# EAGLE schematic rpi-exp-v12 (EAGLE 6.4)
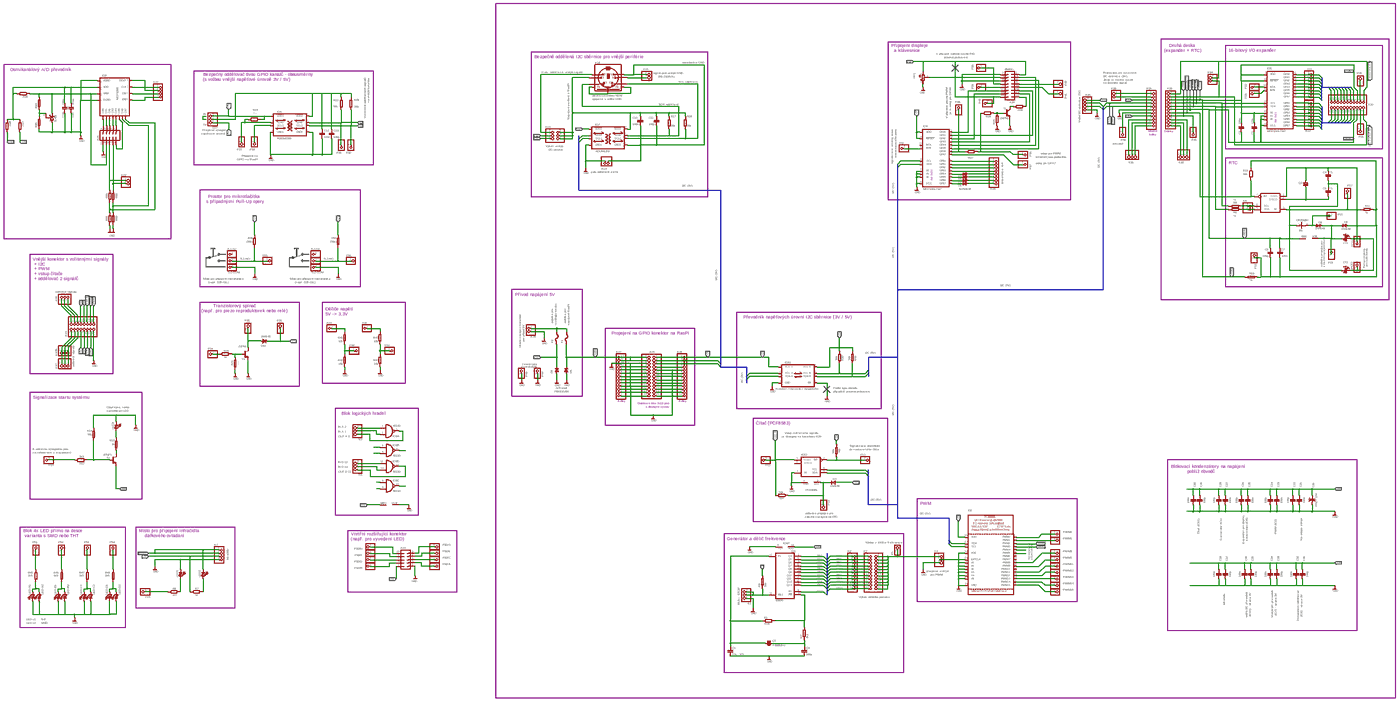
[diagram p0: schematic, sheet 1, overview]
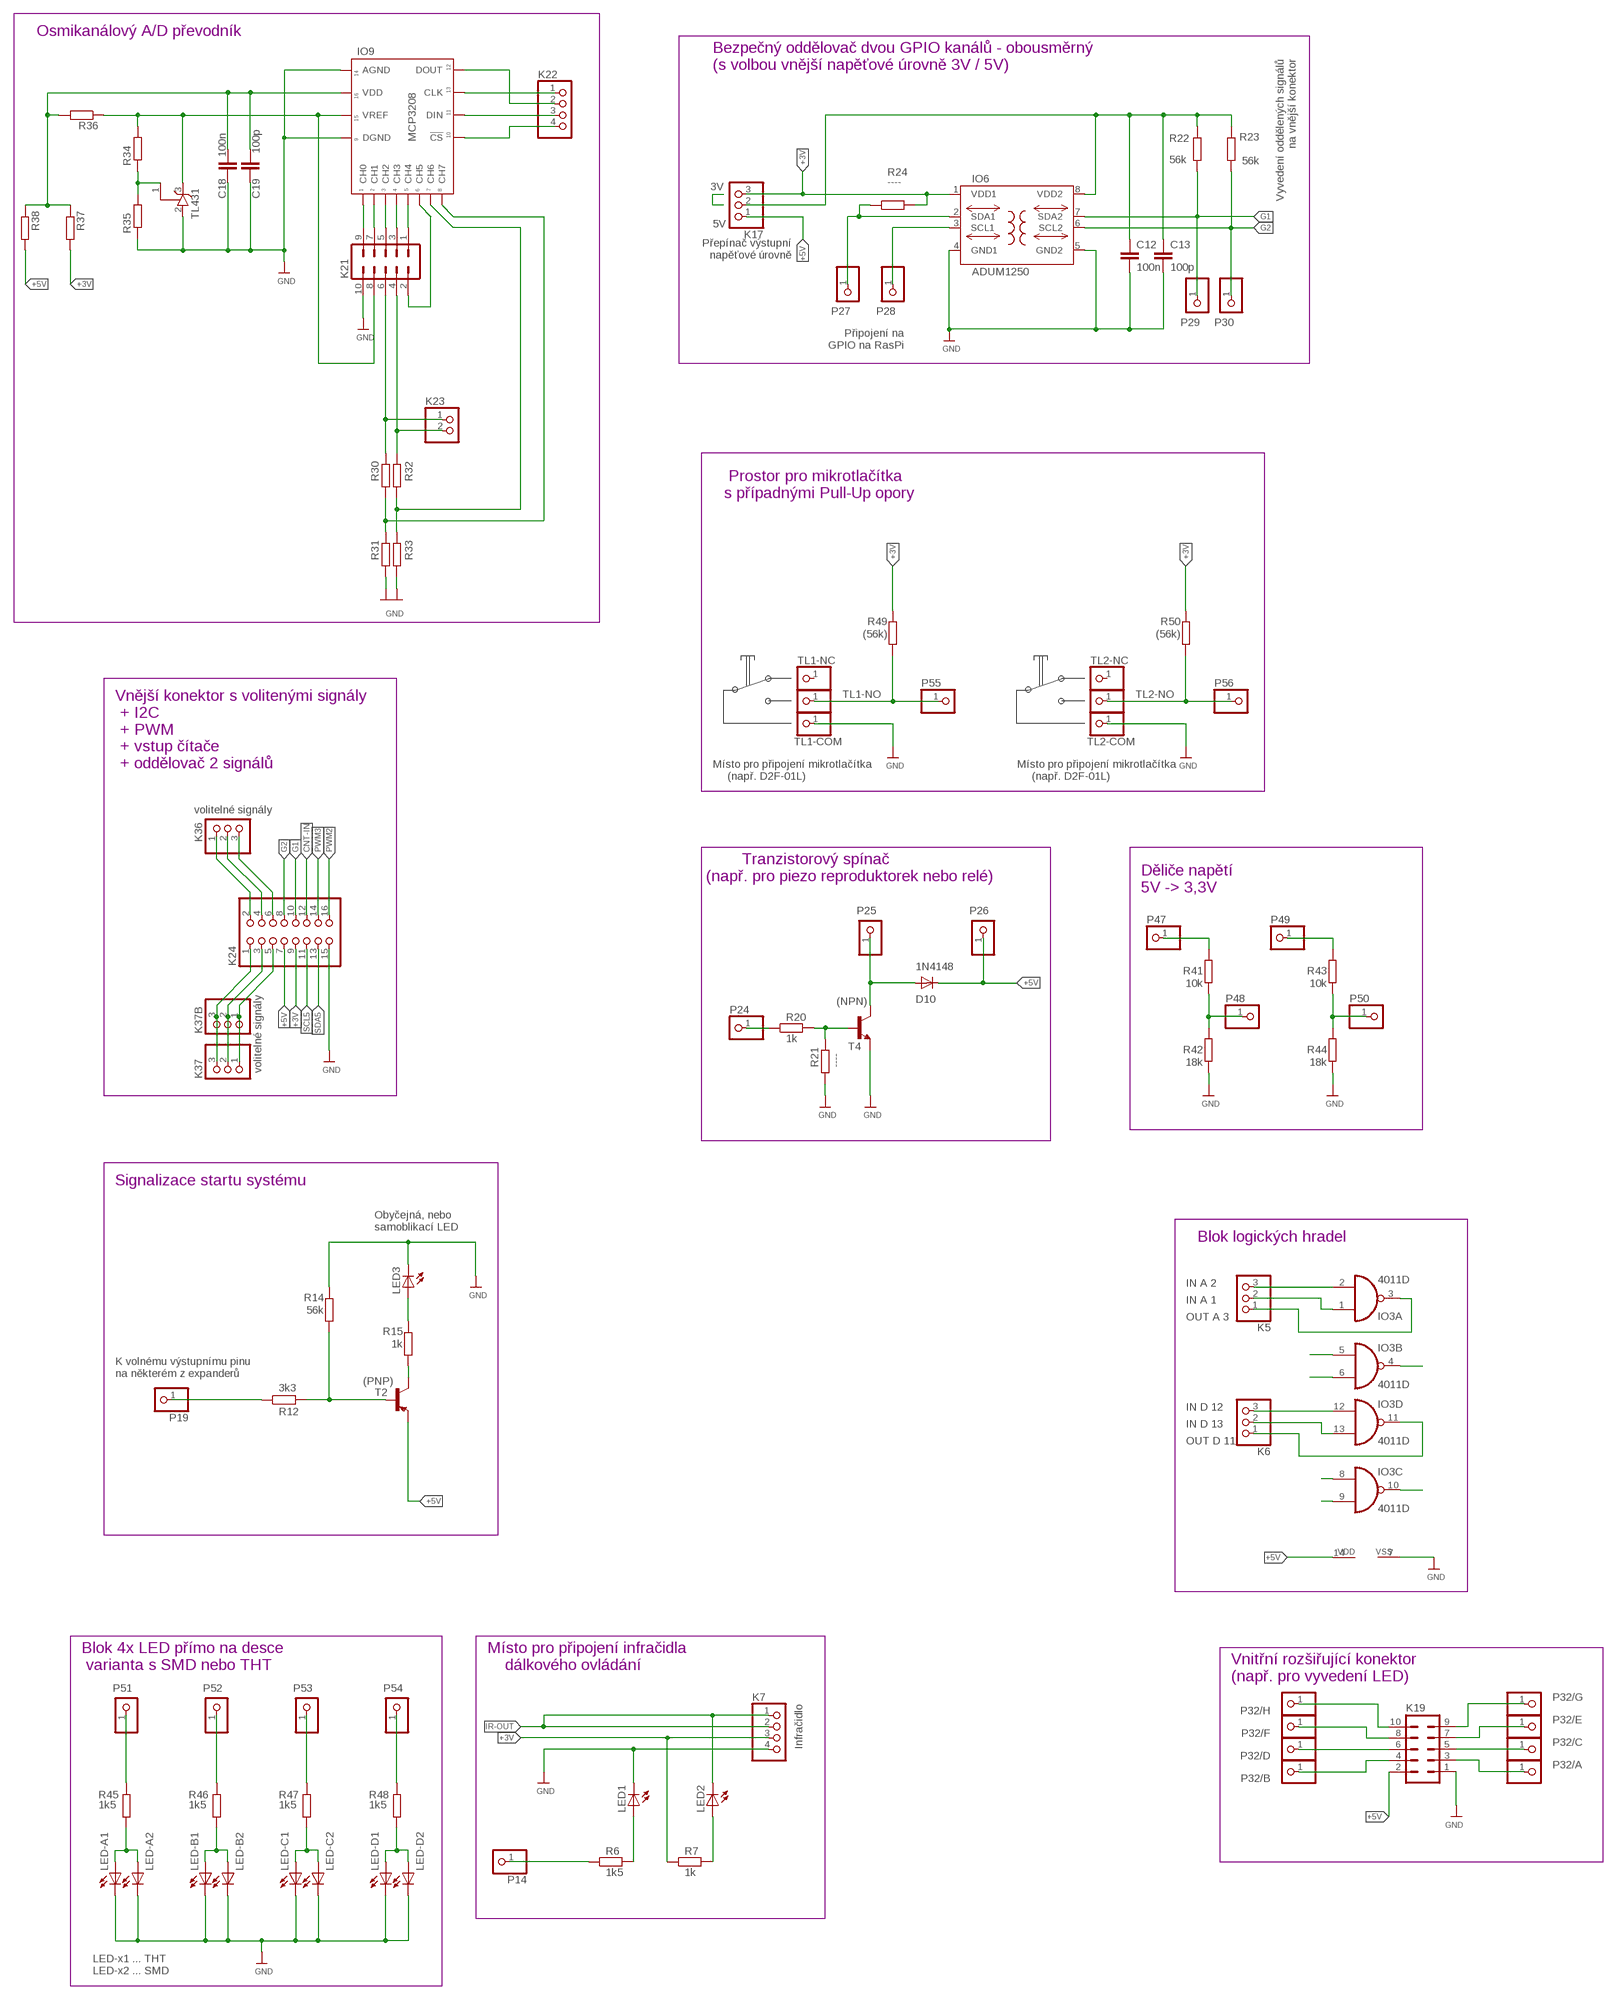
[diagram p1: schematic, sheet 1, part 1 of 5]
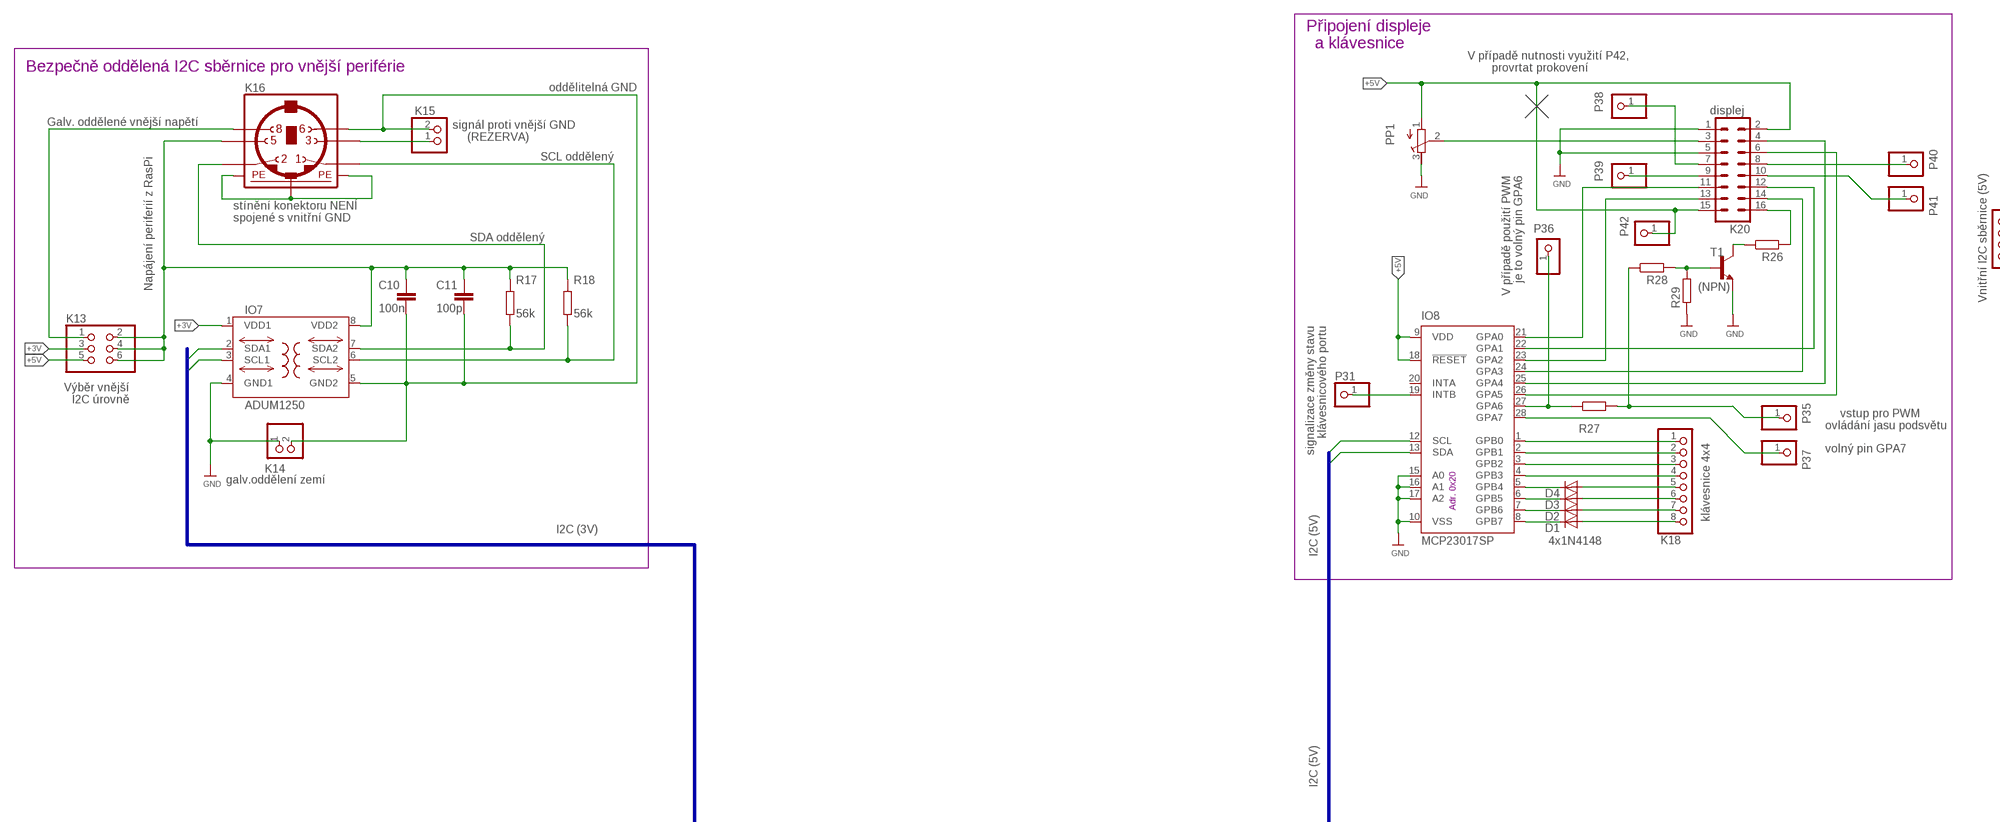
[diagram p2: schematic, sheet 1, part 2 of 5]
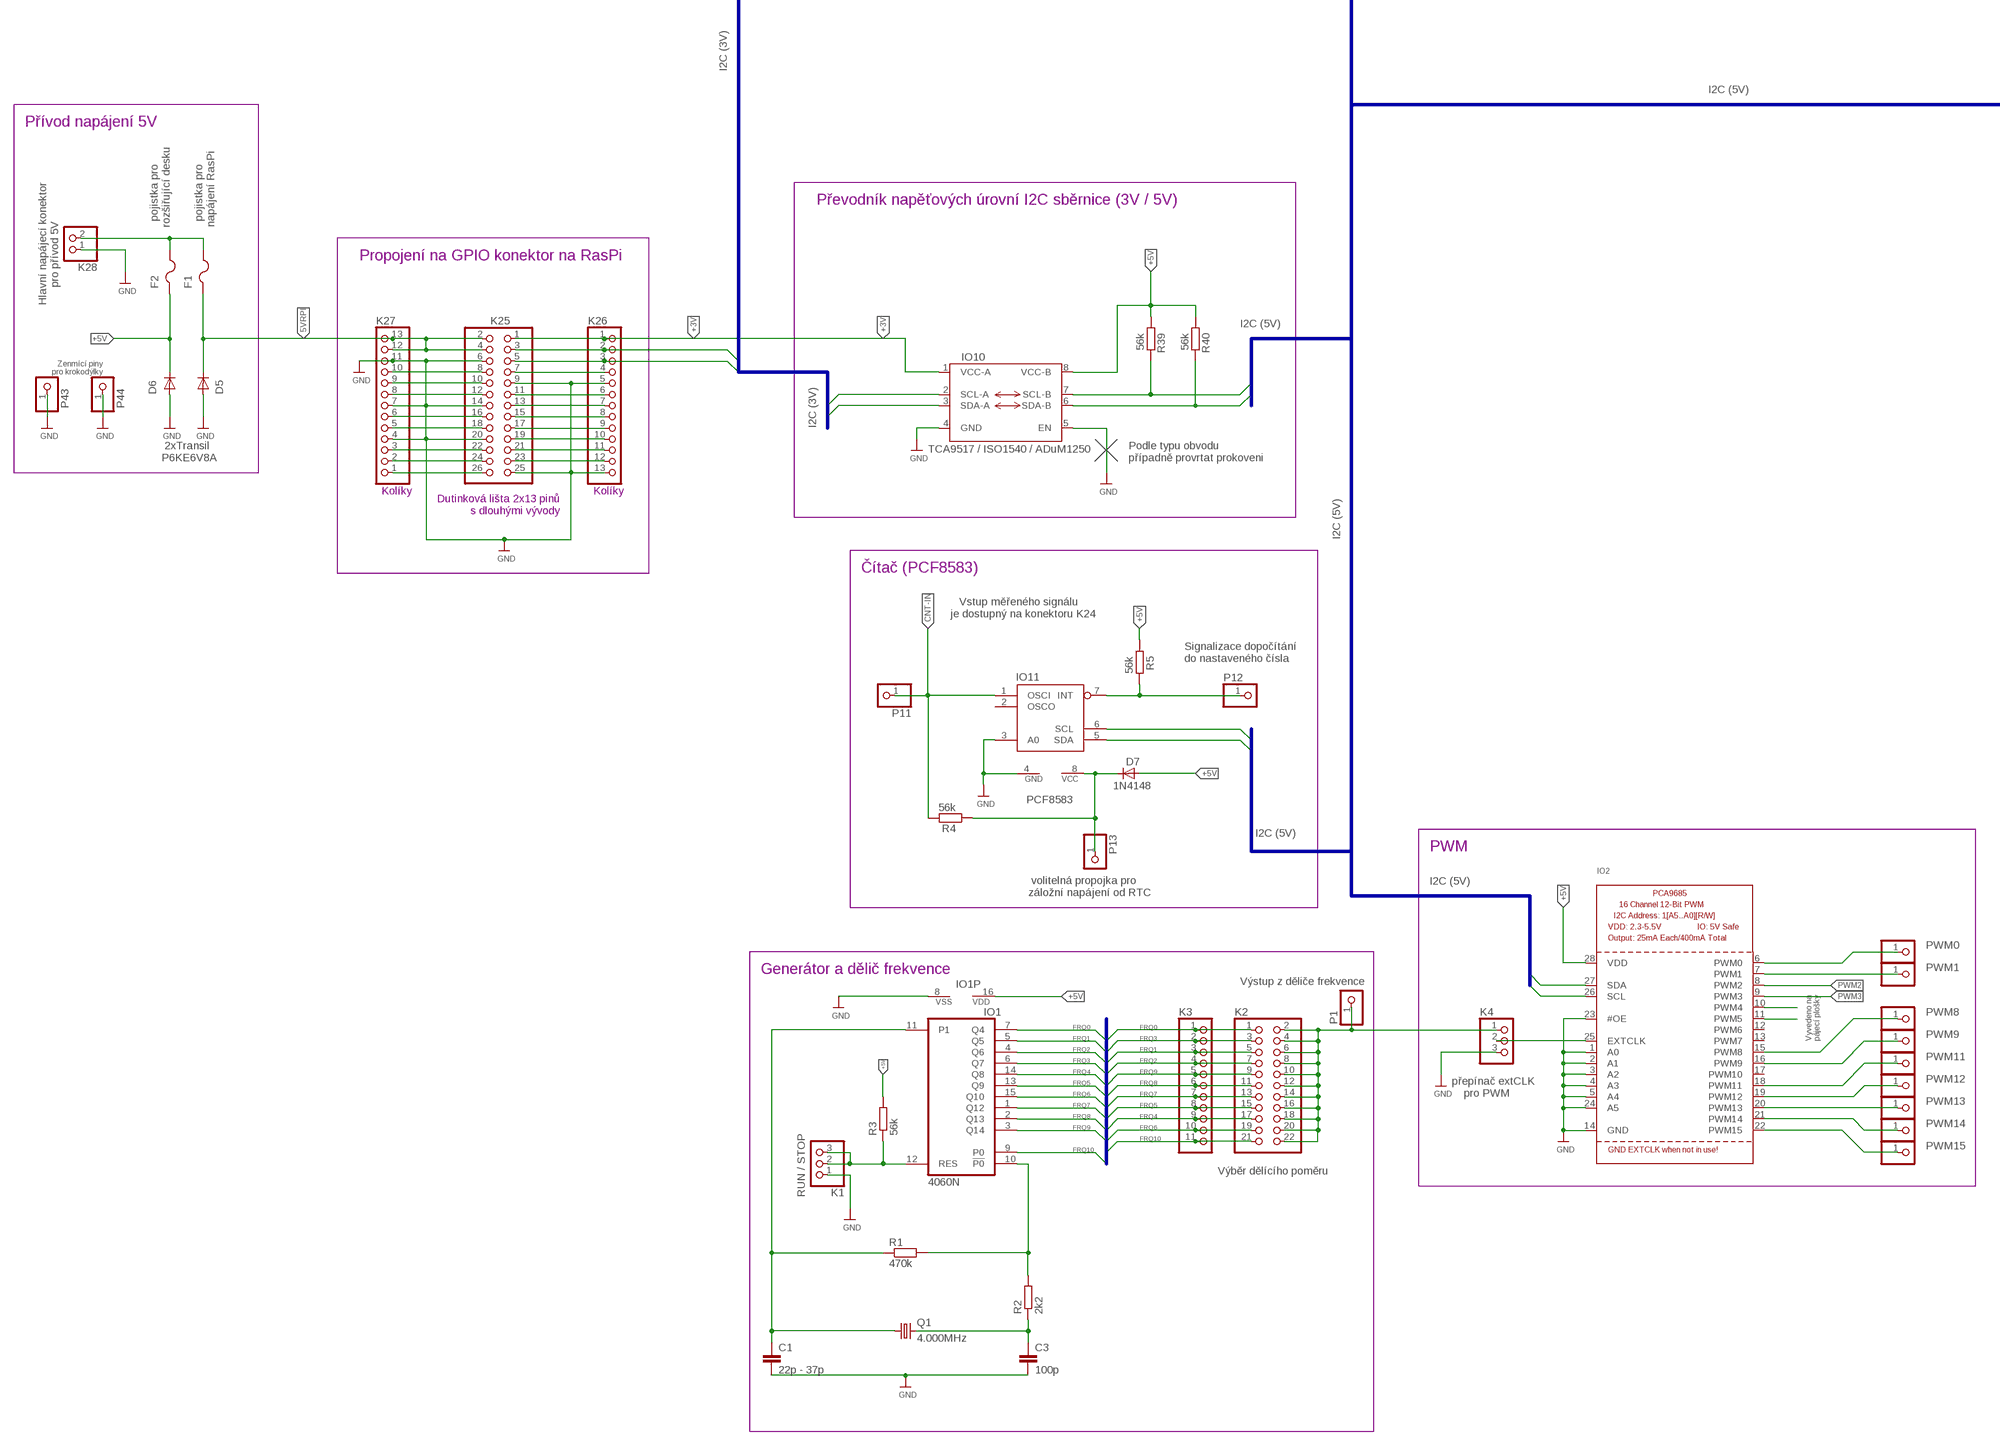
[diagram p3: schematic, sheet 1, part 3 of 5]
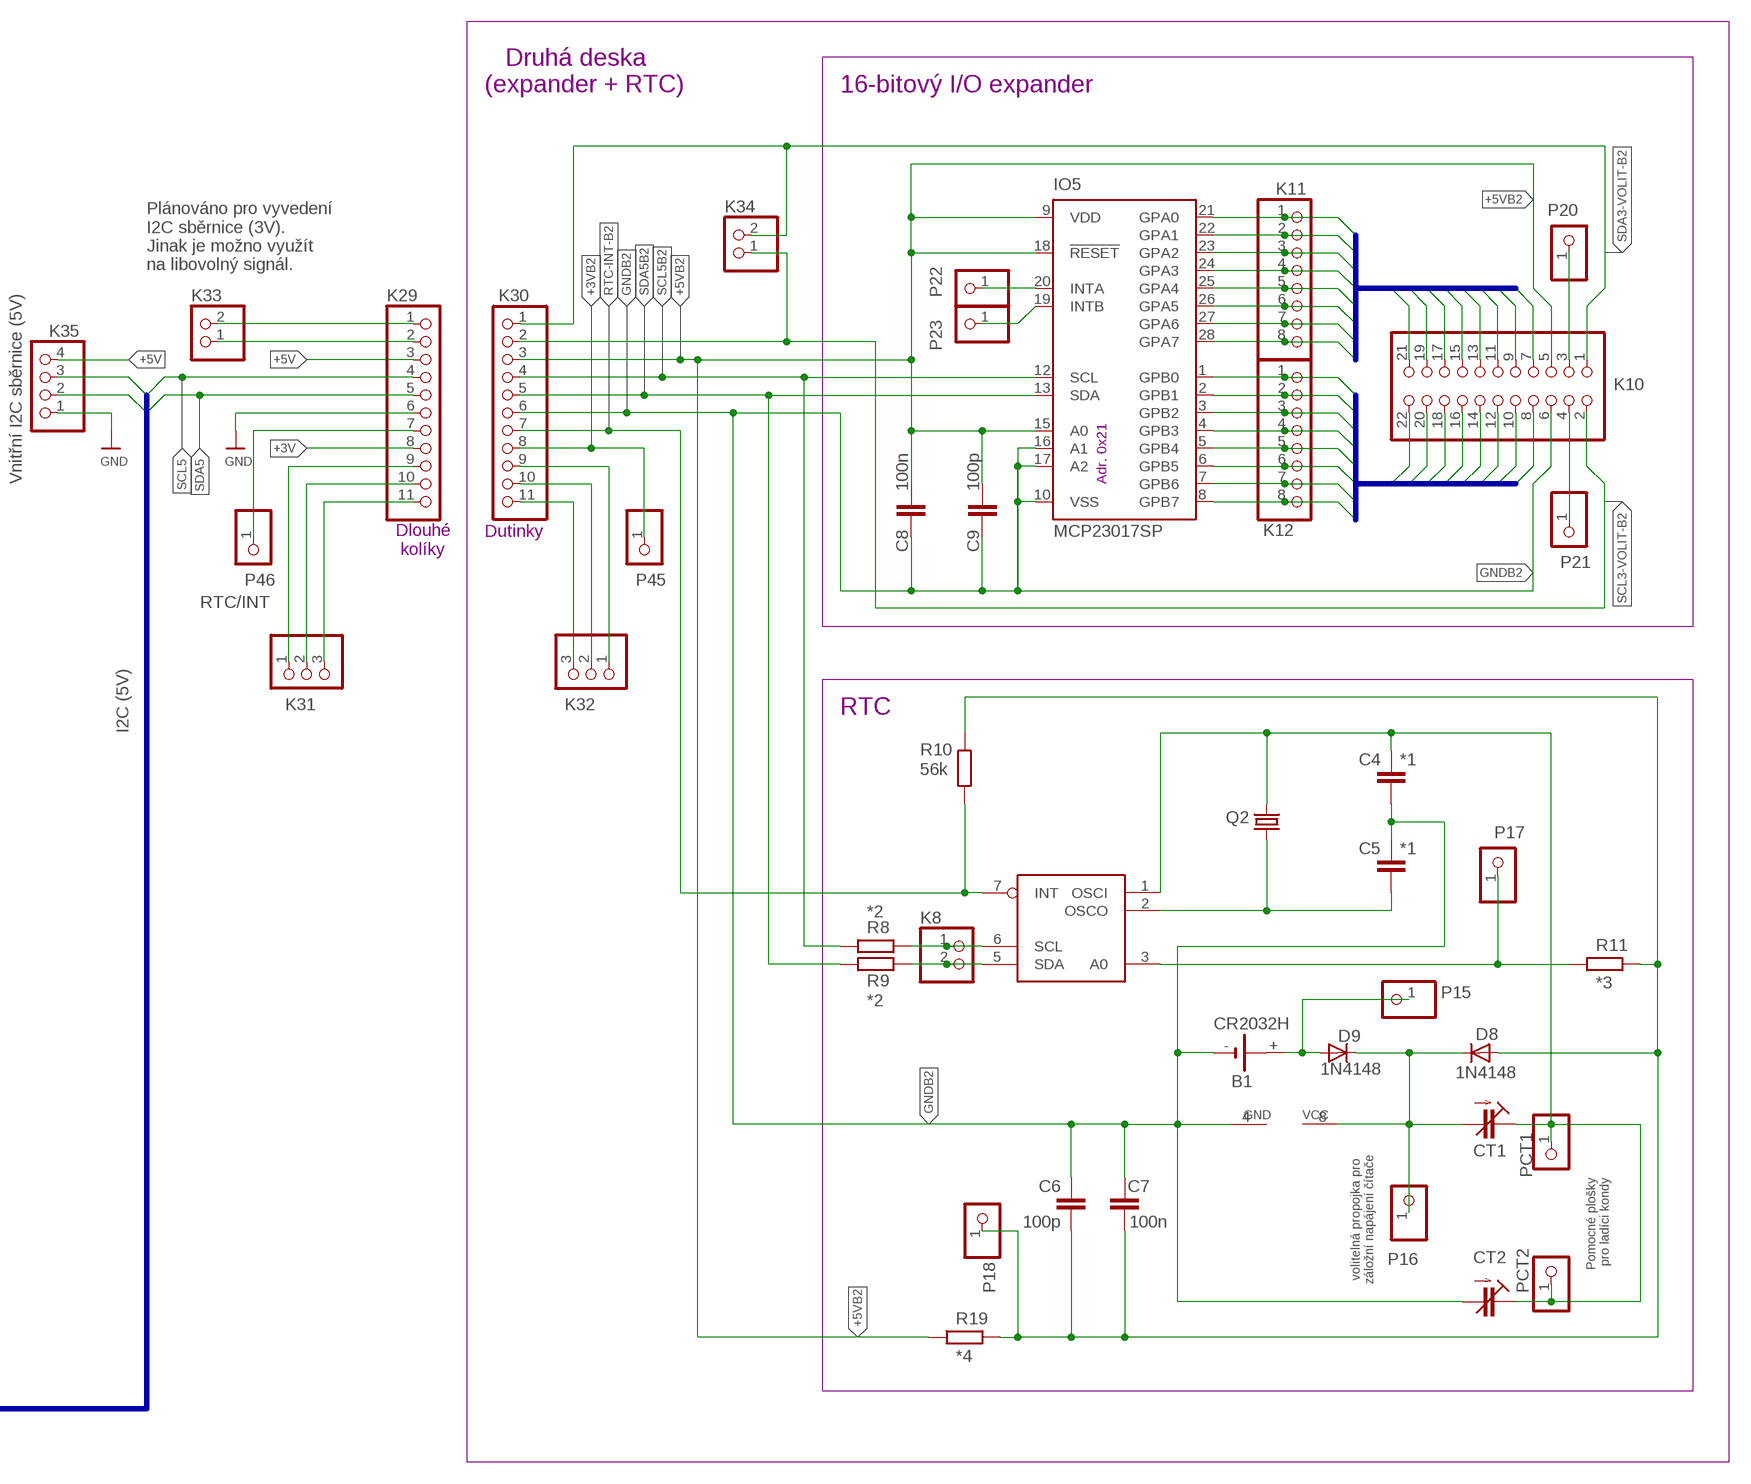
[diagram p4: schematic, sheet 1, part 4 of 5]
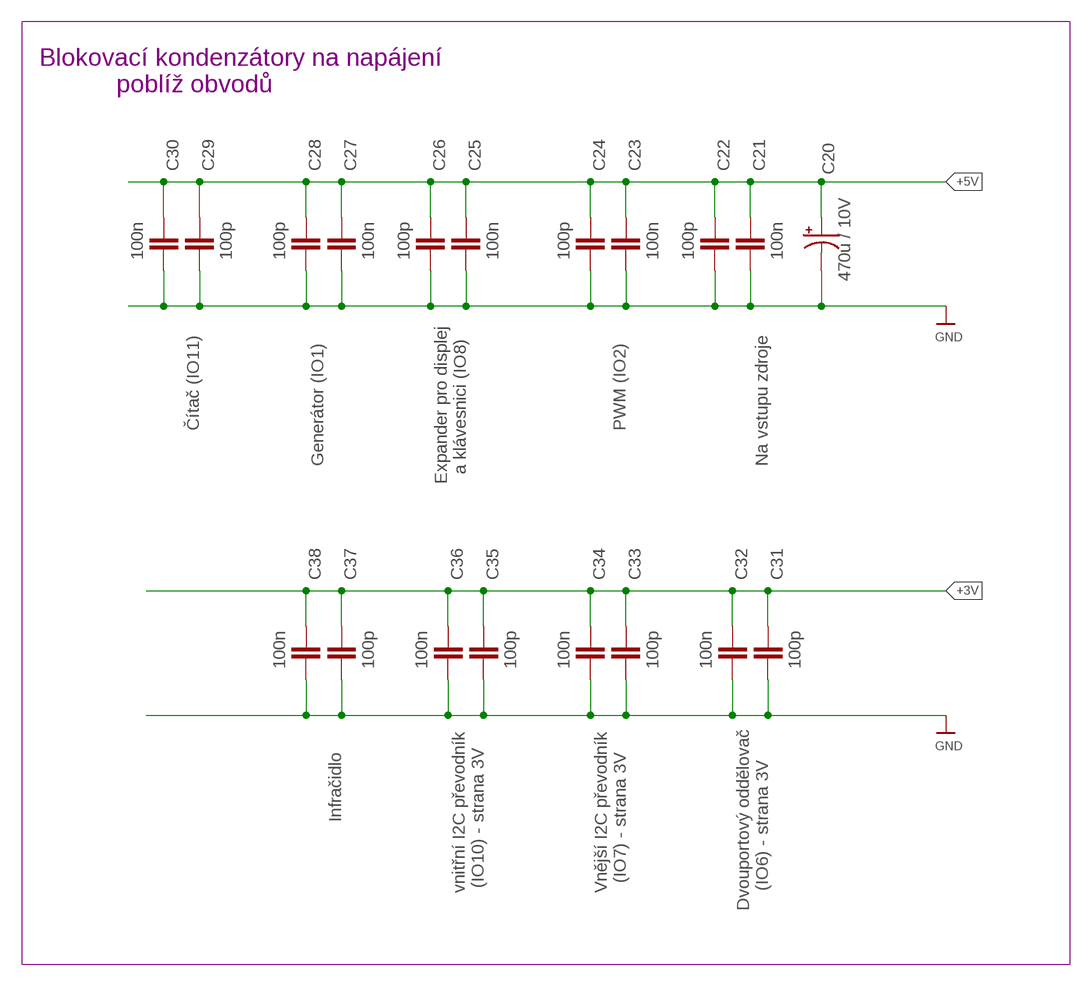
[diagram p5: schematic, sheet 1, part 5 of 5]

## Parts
B1  CR2032H  [CR2032H]
C1  22p - 37p  C-SMD0805  [0805]
C3  100p  C-SMD0805  [0805]
C4  *1  C-SMD0805  [0805]
C5  *1  C-SMD0805  [0805]
C6  100p  C-SMD0805  [0805]
C7  100n  C-SMD0805  [0805]
C8  100n  C-SMD0805  [0805]
C9  100p  C-SMD0805  [0805]
C10  100n  C-SMD0805  [0805]
C11  100p  C-SMD0805  [0805]
C12  100n  C-SMD0805  [0805]
C13  100p  C-SMD0805  [0805]
C18  100n  C-SMD0805  [0805]
C19  100p  C-SMD0805  [0805]
C20  470u / 10V  CPOL-USE5-8.5  [E5-8,5]
C21  100n  C-SMD0805  [0805]
C22  100p  C-SMD0805  [0805]
C23  100n  C-SMD0805  [0805]
C24  100p  C-SMD0805  [0805]
C25  100n  C-SMD0805  [0805]
C26  100p  C-SMD0805  [0805]
C27  100n  C-SMD0805  [0805]
C28  100p  C-SMD0805  [0805]
C29  100p  C-SMD0805  [0805]
C30  100n  C-SMD0805  [0805]
C31  100p  C-SMD0805  [0805]
C32  100n  C-SMD0805  [0805]
C33  100p  C-SMD0805  [0805]
C34  100n  C-SMD0805  [0805]
C35  100p  C-SMD0805  [0805]
C36  100n  C-SMD0805  [0805]
C37  100p  C-SMD0805  [0805]
C38  100n  C-SMD0805  [0805]
CT1  C-TRIMM3040.427  [CTRIM3040.427]
CT2  C-TRIMM3040.427  [CTRIM3040.427]
D1  1N4148  DIODE-SOD106A-R  [SOD106A-R]
D2  1N4148  DIODE-SOD106A-R  [SOD106A-R]
D3  1N4148  DIODE-SOD106A-R  [SOD106A-R]
D4  1N4148  DIODE-SOD106A-R  [SOD106A-R]
D5  P6KE6V8A  1N4004  [DO41-10]
D6  P6KE6V8A  1N4004  [DO41-10]
D7  1N4148  D-SOD-80  [SOD80]
D8  1N4148  D-SOD-80  [SOD80]
D9  1N4148  D-SOD-80  [SOD80]
D10  1N4148  DIODE-SOD106A-R  [SOD106A-R]
F1  PTCFUSE-1812  [1812]
F2  PTCFUSE-1812  [1812]
I04  PCF8583P  [DIL08]
IO1  4060N  [DIL16]
IO2  PCA9685  [TSSOP28]
IO3  4011D  [SO14]
IO5  MCP23017SP  [DIL28-3]
IO6  ADUM1250  [SO8-COOL]
IO7  ADUM1250  [SO8-COOL]
IO8  MCP23017SP  [DIL28-3]
IO9  MCP3208  21298EDIP  [DIP16]
IO10  TCA9517 / ISO1540 / ADuM1250  TCA9517  [SO8-COOL]
IO11  PCF8583P  [DIL08]
K1  PINHD-1X3  [1X03]
K2  PINHD-2X11  [2X11]
K3  PINHD-1X11  [1X11]
K4  PINHD-1X3  [1X03]
K5  PINHD-1X3  [1X03]
K6  PINHD-1X3  [1X03]
K7  PINHD-1X4  [1X04]
K8  PINHD-1X2  [1X02]
K10  PINHD-2X11/90  [2X11/90]
K11  PINHD-1X8  [1X08]
K12  PINHD-1X8  [1X08]
K13  PINHD-2X3  [2X03]
K14  PINHD-1X2  [1X02]
K15  PINHD-1X2  [1X02]
K16  MINI_DIN_6  [M_DIN6]
K17  PINHD-1X3  [1X03]
K18  PINHD-1X8  [1X08]
K19  ML10  [ML10]
K20  ML16  [ML16]
K21  ML10L  [ML10L]
K22  PINHD-1X4  [1X04]
K23  PINHD-1X2  [1X02]
K24  PINHD-2X8/90  [2X08/90]
K25  PINHD-2X13  [2X13]
K26  PINHD-1X13  [1X13]
K27  PINHD-1X13  [1X13]
K28  PINHD-1X2  [1X02]
K29  PINHD-1X11  [1X11]
K30  PINHD-1X11  [1X11]
K31  PINHD-1X3  [1X03]
K32  PINHD-1X3  [1X03]
K33  PINHD-1X2  [1X02]
K34  PINHD-1X2  [1X02]
K35  PINHD-1X4  [1X04]
K36  PINHD-1X3  [1X03]
K37  PINHD-1X3  [1X03]
K37B  PINHD-1X3  [1X03]
LED1  LED3MM  [LED3MM]
LED2  LED3MM  [LED3MM]
LED3  LED5MM  [LED5MM]
LED-A1  LED3MM  [LED3MM]
LED-A2  LEDCHIP-LED0805  [CHIP-LED0805]
LED-B1  LED3MM  [LED3MM]
LED-B2  LEDCHIP-LED0805  [CHIP-LED0805]
LED-C1  LED3MM  [LED3MM]
LED-C2  LEDCHIP-LED0805  [CHIP-LED0805]
LED-D1  LED3MM  [LED3MM]
LED-D2  LEDCHIP-LED0805  [CHIP-LED0805]
P1  HEADER-1X1  [1X01_OVAL]
P11  HEADER-1X1  [1X01_OVAL]
P12  HEADER-1X1  [1X01_OVAL]
P13  HEADER-1X1  [1X01_OVAL]
P14  HEADER-1X1  [1X01_OVAL]
P15  HEADER-1X1  [1X01_OVAL]
P16  HEADER-1X1  [1X01_OVAL]
P17  HEADER-1X1  [1X01_OVAL]
P18  HEADER-1X1  [1X01_OVAL]
P19  HEADER-1X1  [1X01_OVAL]
P20  HEADER-1X1  [1X01_OVAL]
P21  HEADER-1X1  [1X01_OVAL]
P22  HEADER-1X1  [1X01_OVAL]
P23  HEADER-1X1  [1X01_OVAL]
P24  HEADER-1X1  [1X01_OVAL]
P25  HEADER-1X1  [1X01_OVAL]
P26  HEADER-1X1  [1X01_OVAL]
P27  HEADER-1X1  [1X01_OVAL]
P28  HEADER-1X1  [1X01_OVAL]
P29  HEADER-1X1  [1X01_OVAL]
P30  HEADER-1X1  [1X01_OVAL]
P31  HEADER-1X1  [1X01_OVAL]
P32/A  HEADER-1X1  [1X01_OVAL]
P32/B  HEADER-1X1  [1X01_OVAL]
P32/C  HEADER-1X1  [1X01_OVAL]
P32/D  HEADER-1X1  [1X01_OVAL]
P32/E  HEADER-1X1  [1X01_OVAL]
P32/F  HEADER-1X1  [1X01_OVAL]
P32/G  HEADER-1X1  [1X01_OVAL]
P32/H  HEADER-1X1  [1X01_OVAL]
P35  HEADER-1X1  [1X01_OVAL]
P36  HEADER-1X1  [1X01_OVAL]
P37  HEADER-1X1  [1X01_OVAL]
P38  HEADER-1X1  [1X01_OVAL]
P39  HEADER-1X1  [1X01_OVAL]
P40  PINHD-1X1  [1X01]
P41  PINHD-1X1  [1X01]
P42  HEADER-1X1  [1X01_OVAL]
P43  HEADER-1X1  [1X01_OVAL]
P44  HEADER-1X1  [1X01_OVAL]
P45  HEADER-1X1  [1X01_OVAL]
P46  HEADER-1X1  [1X01_OVAL]
P47  HEADER-1X1  [1X01_OVAL]
P48  HEADER-1X1  [1X01_OVAL]
P49  HEADER-1X1  [1X01_OVAL]
P50  HEADER-1X1  [1X01_OVAL]
P51  HEADER-1X1  [1X01_OVAL]
P52  HEADER-1X1  [1X01_OVAL]
P53  HEADER-1X1  [1X01_OVAL]
P54  HEADER-1X1  [1X01_OVAL]
P55  HEADER-1X1  [1X01_OVAL]
P56  HEADER-1X1  [1X01_OVAL]
PCT1  HEADER-1X1  [1X01_OVAL]
PCT2  HEADER-1X1  [1X01_OVAL]
PP1  R-TRIMM3296Y  [RTRIM3296Y]
PWM0  HEADER-1X1  [1X01_OVAL]
PWM1  HEADER-1X1  [1X01_OVAL]
PWM8  HEADER-1X1  [1X01_OVAL]
PWM9  HEADER-1X1  [1X01_OVAL]
PWM11  HEADER-1X1  [1X01_OVAL]
PWM12  HEADER-1X1  [1X01_OVAL]
PWM13  HEADER-1X1  [1X01_OVAL]
PWM14  HEADER-1X1  [1X01_OVAL]
PWM15  HEADER-1X1  [1X01_OVAL]
Q1  4.000MHz  CRYSTALHC49U-V  [HC49U-V]
Q2  CRYSTALTC26V  [TC26V]
R1  470k  R-EU_M0805  [M0805]
R2  2k2  R-EU_M0805  [M0805]
R3  56k  R-EU_M0805  [M0805]
R4  56k  R-EU_M0805  [M0805]
R5  56k  R-EU_M0805  [M0805]
R6  1k5  R-EU_M0805  [M0805]
R7  1k  R-EU_M0805  [M0805]
R8  *2  R-EU_M0805  [M0805]
R9  *2  R-EU_M0805  [M0805]
R10  56k  R-EU_M0805  [M0805]
R11  *3  R-EU_M0805  [M0805]
R12  3k3  R-EU_M0805  [M0805]
R14  56k  R-EU_M0805  [M0805]
R15  1k  R-EU_M0805  [M0805]
R17  56k  R-EU_M0805  [M0805]
R18  56k  R-EU_M0805  [M0805]
R19  *4  R-EU_M0805  [M0805]
R20  1k  R-EU_M0805  [M0805]
R21  ----  R-EU_M0805  [M0805]
R22  56k  R-EU_M0805  [M0805]
R23  56k  R-EU_M0805  [M0805]
R24  ----  R-EU_M0805  [M0805]
R26  R-EU_M0805  [M0805]
R27  R-EU_M0805  [M0805]
R28  R-EU_M0805  [M0805]
R29  R-EU_M0805  [M0805]
R30  R-EU_M0805  [M0805]
R31  R-EU_M0805  [M0805]
R32  R-EU_M0805  [M0805]
R33  R-EU_M0805  [M0805]
R34  R-EU_M0805  [M0805]
R35  R-EU_M0805  [M0805]
R36  R-EU_M0805  [M0805]
R37  R-EU_M0805  [M0805]
R38  R-EU_M0805  [M0805]
R39  56k  R-EU_M0805  [M0805]
R40  56k  R-EU_M0805  [M0805]
R41  10k  R-EU_M0805  [M0805]
R42  18k  R-EU_M0805  [M0805]
R43  10k  R-EU_M0805  [M0805]
R44  18k  R-EU_M0805  [M0805]
R45  1k5  R-EU_M0805  [M0805]
R46  1k5  R-EU_M0805  [M0805]
R47  1k5  R-EU_M0805  [M0805]
R48  1k5  R-EU_M0805  [M0805]
R49  (56k)  R-EU_M0805  [M0805]
R50  (56k)  R-EU_M0805  [M0805]
STAB1  TL431  [TO92]
T1  (NPN)  2N2222  [TO92-EBC-OVAL]
T2  (PNP)  2N3906  [TO92]
T4  (NPN)  2N2222  [TO92-EBC-OVAL]
TL1-COM  HEADER-1X1  [1X01_OVAL]
TL1-NC  HEADER-1X1  [1X01_OVAL]
TL1-NO  HEADER-1X1  [1X01_OVAL]
TL2-COM  HEADER-1X1  [1X01_OVAL]
TL2-NC  HEADER-1X1  [1X01_OVAL]
TL2-NO  HEADER-1X1  [1X01_OVAL]

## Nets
5VRPI: D5.C F1.1 K25.2 K25.4 K27.12 K27.13
4011-4: IO3.4(B:O)
4011-5: IO3.5(B:I0)
4011-6: IO3.6(B:I1)
4011-8: IO3.8(C:I0)
4011-9: IO3.9(C:I1)
4011-10: IO3.10(C:O)
+3V: C31.1 C32.1 C33.1 C34.1 C35.1 C36.1 C37.1 C38.1 IO6.1(VDD1) IO7.1(VDD1) IO10.1(VCC-A) K7.3 K13.3 K17.3 K24.9 K25.1 K26.1 K29.8 R7.1 R24.2 R37.2 R49.2 R50.2
+3VB2: K30.8 P45.1
+5V: C20.+ C21.1 C22.1 C23.1 C24.1 C25.1 C26.1 C27.1 C28.1 C29.1 C30.1 D6.C D7.2(A) D10.C F2.1 IO1.16(VDD) IO2.28(VDD) IO3.14(P:VDD) IO8.9(VDD) IO8.18(!RESET) IO10.8(VCC-B) K13.5 K17.1 K19.2 K20.2 K20.15 K24.7 K29.3 K35.4 P26.1 P42.1 PP1.1(E) R3.2 R5.1 R38.2 R39.1 R40.1 T2.3(E)
+5VB2: C8.2 C9.1 IO5.9(VDD) IO5.15(A0) IO5.18(!RESET) K10.5 K30.3 R19.1
AD-VCC: C18.2 C19.2 IO9.P$16(VDD) R36.2 R37.1 R38.1
ADC0: IO9.P$1(CH0) K21.9
ADC1: IO9.P$2(CH1) K21.7
ADC2: IO9.P$3(CH2) K21.5
ADC3: IO9.P$4(CH3) K21.3
ADC4: IO9.P$5(CH4) K21.1
ADC5: IO9.P$6(CH5) K21.2
ADC6: IO9.P$7(CH6) R32.1 R33.2
ADC7: IO9.P$8(CH7) R30.1 R31.2
ADC-D6: K21.4 K23.2 R32.2
ADC-D7: K21.6 K23.1 R30.2
BCKUP+: B1.+ D9.2(A) P15.1
BCKUP-CNT: D7.1(C) IO11.8(VCC) P13.1 R4.1
CNT-IN: IO11.1(OSCI) K24.12 P11.1 R4.2
CNT-INT: IO11.7(INT) P12.1 R5.2
DIS-KONTR: K20.3 PP1.2(S)
FRQ0: IO1.7(Q4) K2.1 K3.1
FRQ1: IO1.5(Q5) K2.5 K3.3
FRQ2: IO1.4(Q6) K2.7 K3.4
FRQ3: IO1.6(Q7) K2.3 K3.2
FRQ4: IO1.14(Q8) K2.17 K3.9
FRQ5: IO1.13(Q9) K2.15 K3.8
FRQ6: IO1.15(Q10) K2.19 K3.10
FRQ7: IO1.1(Q12) K2.13 K3.7
FRQ8: IO1.2(Q13) K2.11 K3.6
FRQ9: IO1.3(Q14) K2.9 K3.5
FRQ10: IO1.9(P0) K2.21 K3.11
G1: IO6.7(SDA2) K24.10 P29.1 R22.2
G2: IO6.6(SCL2) K24.8 P30.1 R23.2
GND: C1.2 C3.2 C12.2 C13.2 C18.1 C19.1 C20.- C21.2 C22.2 C23.2 C24.2 C25.2 C26.2 C27.2 C28.2 C29.2 C30.2 C31.2 C32.2 C33.2 C34.2 C35.2 C36.2 C37.2 C38.2 D5.A D6.A IO1.8(VSS) IO2.1(A0) IO2.2(A1) IO2.3(A2) IO2.4(A3) IO2.5(A4) IO2.14(GND) IO2.23(#OE) IO2.24(A5) IO3.7(P:VSS) IO6.4(GND1) IO6.5(GND2) IO7.4(GND1) IO8.10(VSS) IO8.15(A0) IO8.16(A1) IO8.17(A2) IO9.P$9(DGND) IO9.P$14(AGND) IO10.4(GND) IO10.5(EN) IO11.3(A0) IO11.4(GND) K1.1 K4.3 K7.4 K14.1 K19.1 K20.1 K20.5 K21.10 K24.15 K25.6 K25.9 K25.14 K25.20 K25.25 K26.5 K26.13 K27.4 K27.7 K27.11 K28.1 K29.6 K35.1 LED1.K(C) LED3.K(C) LED-A1.K(C) LED-A2.C LED-B1.K(C) LED-B2.C LED-C1.K(C) LED-C2.C LED-D1.K(C) LED-D2.C P43.1 P44.1 PP1.3(A) R14.1 R21.1 R29.1 R31.1 R33.1 R35.1 R42.1 R44.1 STAB1.2(A) T1.E T4.E TL1-COM.1 TL2-COM.1
GND2: C10.2 C11.2 IO7.5(GND2) K14.2 K15.2 K16.6
GNDB2: B1.- C4.1 C5.2 C6.2 C7.2 C8.1 C9.2 CT2.2(A) I04.4(GND) IO5.10(VSS) IO5.16(A1) IO5.17(A2) K10.6 K30.6
GPA0: IO5.21(GPA0) K10.7 K11.1
GPA1: IO5.22(GPA1) K10.9 K11.2
GPA2: IO5.23(GPA2) K10.11 K11.3
GPA3: IO5.24(GPA3) K10.13 K11.4
GPA4: IO5.25(GPA4) K10.15 K11.5
GPA5: IO5.26(GPA5) K10.17 K11.6
GPA6: IO5.27(GPA6) K10.19 K11.7
GPA7: IO5.28(GPA7) K10.21 K11.8
GPB0: IO5.1(GPB0) K10.22 K12.1
GPB1: IO5.2(GPB1) K10.20 K12.2
GPB2: IO5.3(GPB2) K10.18 K12.3
GPB3: IO5.4(GPB3) K10.16 K12.4
GPB4: IO5.5(GPB4) K10.14 K12.5
GPB5: IO5.6(GPB5) K10.12 K12.6
GPB6: IO5.7(GPB6) K10.10 K12.7
GPB7: IO5.8(GPB7) K10.8 K12.8
INA1: IO3.1(A:I0) K5.2
INA2: IO3.2(A:I1) K5.3
IND12: IO3.12(D:I0) K6.3
IND13: IO3.13(D:I1) K6.2
IR-OUT: K7.1 K7.2 LED2.K(C)
K24-1: K24.1 K37.3 K37B.3
K24-2: K24.2 K36.1
K24-3: K24.3 K37.2 K37B.2
K24-4: K24.4 K36.2
K24-5: K24.5 K37.1 K37B.1
K24-6: K24.6 K36.3
LED-A: LED-A1.A LED-A2.A R45.2
LED-B: LED-B1.A LED-B2.A R46.2
LED-C: LED-C1.A LED-C2.A R47.2
LED-D: LED-D1.A LED-D2.A R48.2
LED-PIN51: P51.1 R45.1
LED-PIN52: P52.1 R46.1
LED-PIN53: P53.1 R47.1
LED-PIN54: P54.1 R48.1
N$1: IO8.1(GPB0) K18.1
N$2: IO8.2(GPB1) K18.2
N$3: IO8.3(GPB2) K18.3
N$4: IO8.4(GPB3) K18.4
N$5: D4.C IO8.5(GPB4)
N$6: D4.A K18.5
N$7: D3.C IO8.6(GPB5)
N$8: D3.A K18.6
N$9: D2.C IO8.7(GPB6)
N$10: D2.A K18.7
N$11: D1.C IO8.8(GPB7)
N$12: D1.A K18.8
N$13: K25.23 K26.12
N$14: P47.1 R41.2
N$15: K29.9 K31.1
N$17: K25.21 K26.11
N$18: CT1.2(A) D8.1(C) D9.1(C) I04.8(VCC) P16.1
N$19: K25.19 K26.10
N$20: I04.6(SCL) K8.1 R8.2
N$21: K25.13 K26.7
N$22: IO8.21(GPA0) K20.11
N$23: IO8.22(GPA1) K20.12
N$24: IO8.23(GPA2) K20.13
N$25: IO8.24(GPA3) K20.14
N$26: K25.7 K26.4
N$27: K29.11 K31.3
N$28: IO8.25(GPA4) K20.4
N$29: I04.5(SDA) K8.2 R9.2
N$30: IO8.26(GPA5) K20.6
N$32: K30.9 K32.1
N$33: IO8.27(GPA6) P36.1 R27.1
N$34: P35.1 R27.2 R28.1
N$35: R26.1 T1.C
N$36: K20.16 R26.2
N$37: IO7.6(SCL2) K16.1 R18.2
N$38: K30.11 K32.3
N$40: I04.3(A0) P17.1 R11.1
N$41: K13.1 K16.8
N$43: LED3.A R15.1
N$47: K19.9 P32/G.1
N$48: K19.7 P32/E.1
N$49: K19.5 P32/C.1
N$50: K19.3 P32/A.1
N$51: P48.1 R41.1 R42.2
N$58: K19.4 P32/B.1
N$59: K19.6 P32/D.1
N$61: C1.1 IO1.11(P1) Q1.1 R1.1
N$62: IO1.10(!P0) R1.2 R2.2
N$64: C3.1 Q1.2 R2.1
N$72: IO8.28(GPA7) P37.1
N$79: R12.2 R14.2 T2.2(B)
N$81: R15.2 T2.1(C)
N$82: K25.11 K26.6
N$83: P19.1 R12.1
N$84: K25.15 K26.8
N$85: K25.17 K26.9
N$86: K19.10 P32/H.1
N$87: K25.8 K27.10
N$88: K25.10 K27.9
N$89: K20.8 P40.1
N$90: K25.16 K27.6
N$91: K25.12 K27.8
N$92: K25.24 K27.2
N$93: K25.22 K27.3
N$94: K25.26 K27.1
N$95: K25.18 K27.5
N$96: K20.10 P41.1
N$97: K20.9 P39.1
N$98: K20.7 P38.1
N$103: K19.8 P32/F.1
N$105: IO7.7(SDA2) K16.2 R17.2
N$108: K15.1 K16.3
N$109: K16.SH1(PE1) K16.SH2(PE2) K16.SH3(PE3)
N$111: IO1.12(RES) K1.2 K1.3 R3.1
N$112: D10.A P25.1 T4.C
N$113: R20.2 R21.2 T4.B
N$114: P24.1 R20.1
N$115: IO8.19(INTB) P31.1
N$117: C6.1 C7.1 D8.2(A) P18.1 R10.1 R11.2 R19.2
N$118: IO9.P$10(!CS) K22.4
N$119: LED2.A R7.2
N$120: LED1.A R6.2
N$121: P14.1 R6.1
N$136: IO9.P$11(DIN) K22.3
N$140: IO5.20(INTA) P22.1
N$141: IO5.19(INTB) P23.1
N$145: K10.3 P20.1
N$146: K10.4 P21.1
N$151: IO9.P$12(DOUT) K22.2
N$154: IO9.P$13(CLK) K22.1
N$157: P49.1 R43.2
N$160: P50.1 R43.1 R44.2
N$181: R28.2 R29.2 T1.B
N$183: R34.1 R35.2 STAB1.1(R)
OUTA3: IO3.3(A:O) K5.1
OUTD11: IO3.11(D:O) K6.1
PWM0: IO2.6(PWM0) PWM0.1
PWM1: IO2.7(PWM1) PWM1.1
PWM2: IO2.8(PWM2) K24.16
PWM3: IO2.9(PWM3) K24.14
PWM4: IO2.10(PWM4)
PWM5: IO2.11(PWM5)
PWM8: IO2.15(PWM8) PWM8.1
PWM9: IO2.16(PWM9) PWM9.1
PWM11: IO2.18(PWM11) PWM11.1
PWM12: IO2.19(PWM12) PWM12.1
PWM13: IO2.20(PWM13) PWM13.1
PWM14: IO2.21(PWM14) PWM14.1
PWM15: IO2.22(PWM15) PWM15.1
PWM-EXTCLK: IO2.25(EXTCLK) K4.2
PWR+: F1.2 F2.2 K28.2
RPI-G1: IO6.2(SDA1) P27.1 R24.1
RPI-G2: IO6.3(SCL1) P28.1
RTC-INT: K29.7 P46.1
RTC-INT-B2: I04.7(INT) K30.7 R10.2
RTC-P1: C4.2 CT1.1A(E) CT2.1A(E) I04.1(OSCI) PCT1.1 PCT2.1 Q2.2
RTC-P2: C5.1 I04.2(OSCO) Q2.1
SCL3: IO7.3(SCL1) IO10.2(SCL-A) K25.5 K26.3
SCL3-VOLIT: K29.2 K33.1
SCL3-VOLIT-B2: K10.2 K30.2 K34.1
SCL5: IO2.26(SCL) IO8.12(SCL) IO10.7(SCL-B) IO11.6(SCL) K24.11 K29.4 K35.3 R39.2
SCL5B2: IO5.12(SCL) K30.4 R8.1
SDA3: IO7.2(SDA1) IO10.3(SDA-A) K25.3 K26.2
SDA3-VOLIT: K29.1 K33.2
SDA3-VOLIT-B2: K10.1 K30.1 K34.2
SDA5: IO2.27(SDA) IO8.13(SDA) IO10.6(SDA-B) IO11.5(SDA) K24.13 K29.5 K35.2 R40.2
SDA5B2: IO5.13(SDA) K30.5 R9.1
SPOL-FREQ: K2.2 K2.4 K2.6 K2.8 K2.10 K2.12 K2.14 K2.16 K2.18 K2.20 K2.22 K4.1 P1.1
TL1-NO: P55.1 R49.1 TL1-NO.1
TL2-NO: P56.1 R50.1 TL2-NO.1
VDD2: C10.1 C11.1 IO7.8(VDD2) K13.2 K13.4 K13.6 K16.5 R17.1 R18.1
VDD-2: C12.1 C13.1 IO6.8(VDD2) K17.2 R22.1 R23.1
VOLIT2-B1: K29.10 K31.2
VOLIT2-B2: K30.10 K32.2
VREF: IO9.P$15(VREF) K21.8 R34.2 R36.1 STAB1.3(C)
Unconnected: B1.+@1(+) IO2.12(PWM6) IO2.13(PWM7) IO2.17(PWM10) IO8.20(INTA) IO11.2(OSCO) TL1-NC.1 TL2-NC.1

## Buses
SDA5,SCL5
GPA[0..7]
GPB[0..7]
SDA3,SCL3
FRQ[0..10]

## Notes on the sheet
- Připojení displeje
    a klávesnice
- Druhá deska
  (expander + RTC)
- 16-bitový I/O expander
- Bezpečně oddělená I2C sběrnice pro vnější periférie
- V případě nutnosti využití P42,
          provrtat prokovení
- oddělitelná GND
- displej
- Osmikanálový A/D převodník | Galv. oddělené vnější napětí
- Vyvedení oddělených signálů
         na vnější konektor
- signál proti vnější GND
       (REZERVA)
- Bezpečný oddělovač dvou GPIO kanálů - obousměrný
  (s volbou vnější napěťové úrovně 3V / 5V)
- SCL oddělený
- Plánováno pro vyvedení
  I2C sběrnice (3V).
  Jinak je možno využít
  na libovolný signál.
- V případě použití PWM
  je to volný pin GPA6
- stínění konektoru NENÍ
  spojené s vnitřní GND
- SDA oddělený
- 3V
- Napájení periferií z RasPi
- Vnitřní I2C sběrnice (5V) | Adr. 0x21
- 5V
- Přepínač výstupní
  napěťové úrovně
- signalizace změny stavu
    klávesnicového portu
- Dutinky
- Dlouhé
   kolíky
- Výběr vnější
   I2C úrovně
- RTC/INT
- Připojení na
  GPIO na RasPi
- vstup pro PWM
  ovládání jasu podsvětu
- volný pin GPA7 | RTC
- I2C (5V)
- galv.oddělení zemí
- Adr. 0x20
- klávesnice 4x4
- I2C (3V)
- 4x1N4148
- I2C (5V)
- Prostor pro mikrotlačítka
  s případnými Pull-Up opory
- Pomocné plošky
  pro ladíci kondy
- I2C (5V)
- volitelná propojka pro
  záložní napájení čítače
- Vnější konektor s volitenými signály
   + I2C
   + PWM
   + vstup čítače
   + oddělovač 2 signálů
- I2C (3V)
- Místo pro připojení mikrotlačítka
       (např. D2F-01L)
- Místo pro připojení mikrotlačítka
       (např. D2F-01L)
- I2C (5V)
- volitelné signály
- Přívod napájení 5V
- Tranzistorový spínač
   (např. pro piezo reproduktorek nebo relé)
- Děliče napětí
  5V -> 3,3V
- Převodník napěťových úrovní I2C sběrnice (3V / 5V)
- pojistka pro 
  rozšiřující desku
- pojistka pro
  napájení RasPi
- Propojení na GPIO konektor na RasPi
- Hlavní napájecí konektor
        pro přívod 5V
- I2C (5V)
- Zenmící piny
  pro krokodýlky
- volitelné signály
- I2C (3V)
- 2xTransil
   P6KE6V8A
- Podle typu obvodu
  případně provrtat prokoveni
- Signalizace startu systému
- Kolíky
- Dutinková lišta 2x13 pinů
      s dlouhými vývody
- Kolíky
- Obyčejná, nebo 
  samoblikací LED
- Blok logických hradel | I2C (5V)
- Čítač (PCF8583)
- IN A 2
- IN A 1
- OUT A 3
- Vstup měřeného signálu 
  je dostupný na konektoru K24
- Signalizace dopočítání
  do nastaveného čísla
- K volnému výstupnímu pinu
  na některém z expanderů
- IO11
- IN D 12
- IN D 13
- OUT D 11
- Blokovací kondenzátory na napájení
             poblíž obvodů
- PCF8583
- I2C (5V)
- PWM
- I2C (5V)
- volitelná propojka pro
  záložní napájení od RTC
- Čítač (IO11) | PWM (IO2)
- Blok 4x LED přímo na desce
   varianta s SMD nebo THT
- Místo pro připojení infračidla
      dálkového ovládání
- Vnitřní rozšiřující konektor 
  (např. pro vyvedení LED)
- Generátor a dělič frekvence | Generátor (IO1) | Na vstupu zdroje
- Výstup z děliče frekvence
- Expander pro displej
    a klávesnici (IO8)
- Infračidlo
- Vyvedeno na 
  pájecí plošky
- přepínač extCLK
      pro PWM
- Výběr dělícího poměru
- RUN / STOP | Infračidlo
- vnitřní I2C převodník
   (IO10) - strana 3V
- Vnější I2C převodník
    (IO7) - strana 3V
- Dvouportový oddělovač
      (IO6) - strana 3V
- LED-x1 ... THT
  LED-x2 ... SMD

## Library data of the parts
B1 = battery:CR2032H: LI BATTERY Varta
C1 C3-C13 C18 C19 C21-C38 = keramicke kondenzatory SMD:C-SMD: Kondenzátory keramické SMD 50 V
C20 = adafruit:CPOL-US: POLARIZED CAPACITOR, American symbol
CT1 CT2 = rcl:C-TRIMM: Trimm capacitor
D1-D4 D10 = diode:DIODE-: DIODE
D5 D6 = adafruit:1N4004: DIODE
D7-D9 = semicon-smd-ipc:D-: DIODE
F1 F2 = adafruit:PTCFUSE: PTC fuses, resettable thermistors
I04 IO11 = i2c:PCF8583: Clock/calendar with 240 x 8-bit RAM
IO1 = 40xx:4060: 14-stage binary/ripple COUNTER
IO2 = adafruit:PCA9685: PCA9685 - 16 Channel 12-Bit I2C PWM Controller 5.0V tolerant 16 channel, 12-bit I2C PWM controller with 25mA per output (max. 400mA total) Digikey: 568-5931-1-ND
IO3 = 40xx:4011: Quad 2-input NAND
IO5 IO8 = adafruit:MCP23017: http://ww1.microchip.com/downloads/en/DeviceDoc/21952a.pdf Source: http://ww1.microchip.com/downloads/en/DeviceDoc/21952a.pdf
IO6 IO7 = ADuM1250:ADUM1250: Hot Swappable, Dual I2C Isolators Source: http://www.analog.com/static/imported-files/data_sheets/ADUM1250_1251.pdf
IO9 = Microchip-3:21298E
IO10 = tca9517:TCA9517: LEVEL-TRANSLATING I2C BUS REPEATER, TCA9517A Source: http://www.ti.com/product/tca9517
K1 K4-K6 K17 K31 K32 K36 K37 K37B = pinhead:PINHD-1X3: PIN HEADER
K2 K10 = pinhead:PINHD-2X11: PIN HEADER
K3 K29 K30 = pinhead:PINHD-1X11: PIN HEADER
K7 K22 K35 = pinhead:PINHD-1X4: PIN HEADER
K8 K14 K15 K23 K28 K33 K34 = pinhead:PINHD-1X2: PIN HEADER
K11 K12 K18 = pinhead:PINHD-1X8: PIN HEADER
K13 = pinhead:PINHD-2X3: PIN HEADER
K16 = mini_din:MINI_DIN_6
K19 K21 = con-harting-ml:ML10: HARTING; OC_FARNELL: unknown; OC_NEWARK: unknown
K20 = con-ml:ML16: HARTING; OC_FARNELL: unknown; OC_NEWARK: unknown
K24 = pinhead:PINHD-2X8: PIN HEADER
K25 = pinhead:PINHD-2X13: PIN HEADER
K26 K27 = pinhead:PINHD-1X13: PIN HEADER
LED1-LED3 LED-A1 LED-B1 LED-C1 LED-D1 = led:LED: LED
LED-A2 LED-B2 LED-C2 LED-D2 = adafruit:LED: LED
P1 P11-P31 P32/A P32/B P32/C P32/D P32/E P32/F P32/G P32/H P35-P39 P42-P56 PCT1 PCT2 PWM0 PWM1 PWM8 PWM9 PWM11-PWM15 TL1-COM TL1-NC TL1-NO TL2-COM TL2-NC TL2-NO = nonolith:HEADER-1X1: PIN HEADER
P40 P41 = pinhead:PINHD-1X1: PIN HEADER
PP1 = resistor:R-TRIMM: Trimm resistor
Q1 = adafruit:CRYSTAL: CRYSTAL; OC_FARNELL: 1666969; OC_NEWARK: unknown
Q2 = crystal:CRYSTAL: CRYSTAL; OC_FARNELL: unknown; OC_NEWARK: unknown
R1-R12 R14 R15 R17-R24 R39 R40 R45-R50 = resistor:R-EU_: RESISTOR, European symbol
R26-R38 R41-R44 = rcl:R-EU_: RESISTOR, European symbol
STAB1 = stabilizatory:TL431: VOLTAGE REFERENCE
T1 T4 = adafruit:2N2222: NPN TRANSISTOR Big oval pads
T2 = transistor-pnp:2N3906: PNP Transistor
